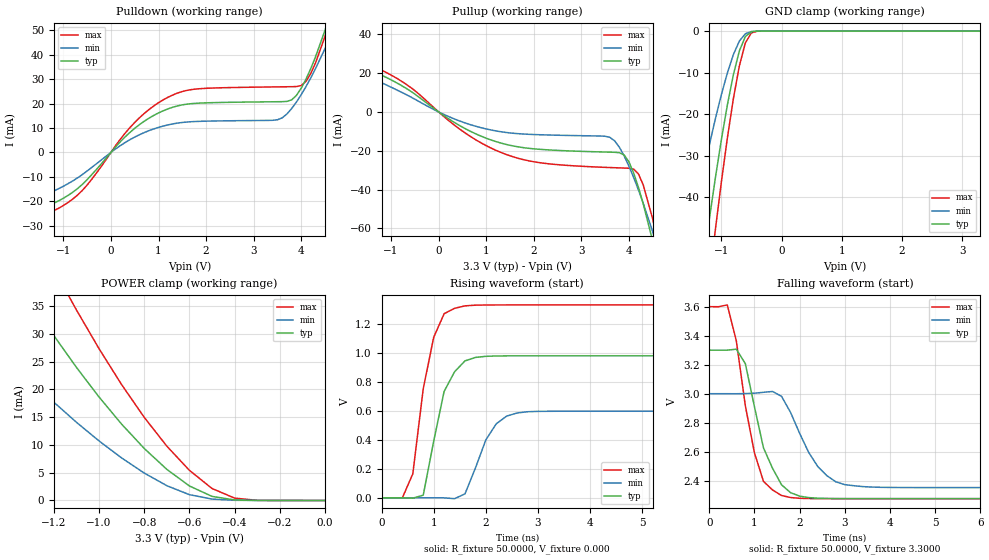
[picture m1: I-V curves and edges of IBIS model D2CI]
| IBIS file t2i.ibs created by s2ibis2 version 1.1
| North Carolina State University Electronics Research Laboratory  1995
[IBIS ver]   2.1
[File name]   d2ci.ibs
[File Rev]   1.0
[Date]   Tuesday, March 28, 2000
[Source]   From silicon level SPICE at TOSHIBA.
[Notes]   This model does not include the values of Package Model
[Disclaimer]   None.
[Copyright]   Copyright(C) TOSHIBA Corp. 1996-2000. All Rights Reserved
|   Component TC260C
[Component]   TC260C
[Manufacturer]   TOSHIBA
[Package]
| variable   typ   min   max
R_pkg   1.00f   NA   NA
L_pkg   1.00fH   NA   NA
C_pkg   1.00fF   NA   NA
[Pin]  signal_name   model_name   R_pin   L_pin   C_pin
IO   IO   D2CI
VDDS   VDDS   POWER
VSS   VSS   GND
| Models and submodels in the file (1): D2CI (I/O)
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|   Model D2CI
[Model]   D2CI
Model_type   I/O
Polarity   Non-Inverting
Vinl   = 0.66V
Vinh   = 2.64V
C_comp   4.3pF   NA   NA
Vmeas = 1.65V
|Variable   typ   min   max
[Voltage range]  3.3   3.0   3.6
[Temperature Range]   25   100   0
[Pullup Reference]   3.3   3.0   3.6
[Pulldown Reference]   0.0   0.0   0.0
[POWER Clamp Reference]   3.3   3.0   3.6
[GND Clamp Reference]   0.0   0.0   0.0
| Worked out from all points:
|   slope of the pulldown table from 0 to 0.495 V, typ, clamps not added: 50.5 ohm
|   slope of the pullup table from 0 to 0.495 V, typ, clamps not added: 63.9 ohm
|   GND clamp passes 1 mA (typ) near -0.57 V on its own axis
|   POWER clamp passes 1 mA (typ) near -0.51 V on its own axis
|   rising waveform, R_fixture 50.0000, V_fixture 0.000: 20-80 % time 378ps typ, 437ps min, 342ps max; typ from 0 V to 0.978 V
|   falling waveform, R_fixture 50.0000, V_fixture 3.3000: 20-80 % time 534ps typ, 652ps min, 440ps max; typ from 3.3 V to 2.28 V
[Pulldown]
| voltage   I(typ)   I(min)   I(max)
-3.3V     -29.37mA   -29.01mA   -32.31mA
-1.9V     -25.53mA   -21.44mA   -28.71mA
-1V       -18.77mA   -13.85mA   -21.76mA
-500mV    -11.12mA   -7.595mA   -13.35mA
500mV     9.878mA    6.294mA    12.28mA
1.3V      18.52mA    11.69mA    23.54mA
3.5V      20.78mA    13.39mA    26.86mA
3.8V      21.56mA    18.01mA    26.94mA
4.1V      30.06mA    26.99mA    29.13mA
4.5V      50.11mA    42.6mA     47.62mA
4.7V      62.45mA    51.64mA    60.99mA
6.6V      227.2mA    181.8mA    250.9mA
[Pullup]
| voltage   I(typ)   I(min)   I(max)
-3.3V     35.88mA    43.25mA    36.87mA
-2.1V     27.55mA    25.61mA    29.91mA
-1.1V     17.77mA    13.9mA     20.3mA
600mV     -9.13mA    -6.021mA   -11.53mA
1.8V      -18.45mA   -11.4mA    -24.67mA
3.6V      -20.71mA   -13.11mA   -28.63mA
3.9V      -22.18mA   -22.69mA   -28.89mA
4.2V      -38.9mA    -40.21mA   -31.94mA
4.3V      -47.34mA   -47.03mA   -37.57mA
4.5V      -66.59mA   -61.78mA   -55.16mA
4.7V      -88.01mA   -77.77mA   -77.42mA
6.6V      -315mA     -263.4mA   -330mA
[GND_clamp]
| voltage   I(typ)   I(min)   I(max)
-3.3V     -292.8mA   -217.8mA   -337.5mA
-1.5V     -77.97mA   -49.07mA   -98.95mA
-1.3V     -55.88mA   -34.36mA   -72.74mA
-1.2V     -45.43mA   -27.57mA   -60.12mA
-1.1V     -35.51mA   -21.22mA   -47.98mA
-900mV    -17.87mA   -10.14mA   -25.85mA
-800mV    -10.56mA   -5.698mA   -16.34mA
-700mV    -4.792mA   -2.412mA   -8.394mA
-600mV    -1.302mA   -649uA     -2.833mA
-500mV    -170.7uA   -108.2uA   -443.3uA
-400mV    -13.58uA   -13.64uA   -33.16uA
3.3V      153.9pA    4.45uA     -1.048nA
[POWER_clamp]
| voltage   I(typ)   I(min)   I(max)
-3.3V     189.1mA    135.9mA    229.2mA
-1.7V     62.57mA    39.06mA    82.98mA
-1.6V     55.54mA    34.4mA     74.31mA
-1.3V     35.75mA    21.56mA    49.45mA
-1.2V     29.69mA    17.7mA     41.7mA
-1.1V     23.96mA    14.08mA    34.3mA
-900mV    13.74mA    7.658mA    20.85mA
-800mV    9.367mA    4.936mA    14.97mA
-600mV    2.612mA    1.048mA    5.42mA
-500mV    737.5uA    251.8uA    2.156mA
-400mV    94.87uA    37.87uA    425.3uA
0V        153.9pA    711.8pA    166.4pA
[Ramp]
| variable   typ   min   max
dV/dt_r   0.5871/0.3313n   0.3581/0.4089n   0.7975/0.3069n
dV/dt_f   0.6138/0.4767n   0.3881/0.6394n   0.7941/0.4120n
R_load = 50.0000
[Rising Waveform]
R_fixture = 50.0000
V_fixture = 0.000
V_fixture_min = 0.000
V_fixture_max = 0.000
| time   V(typ)   V(min)   V(max)
0s        0V         0V         0V
400ps     25.65uV    -34.07uV   -32.64uV
600ps     -2.657mV   19.97uV    165.3mV
800ps     18.2mV     107.4uV    751.5mV
1ns       389.6mV    285.4uV    1.105V
1.2ns     732.7mV    -392.7uV   1.268V
1.4ns     868.1mV    -6.149mV   1.306V
2.2ns     977.4mV    510mV      1.329V
2.6ns     978.4mV    584.5mV    1.329V
10ns      978.5mV    596.8mV    1.329V
[Falling Waveform]
R_fixture = 50.0000
V_fixture = 3.3000
V_fixture_min = 3.0000
V_fixture_max = 3.6000
| time   V(typ)   V(min)   V(max)
0s        3.3V       3V         3.6V
400ps     3.3V       3V         3.612V
600ps     3.307V     3V         3.364V
800ps     3.207V     3.001V     2.916V
1ns       2.911V     3.003V     2.594V
1.2ns     2.627V     3.01V      2.396V
1.6ns     2.372V     2.982V     2.299V
2.4ns     2.28V      2.499V     2.277V
3ns       2.277V     2.373V     2.276V
10ns      2.277V     2.353V     2.276V
